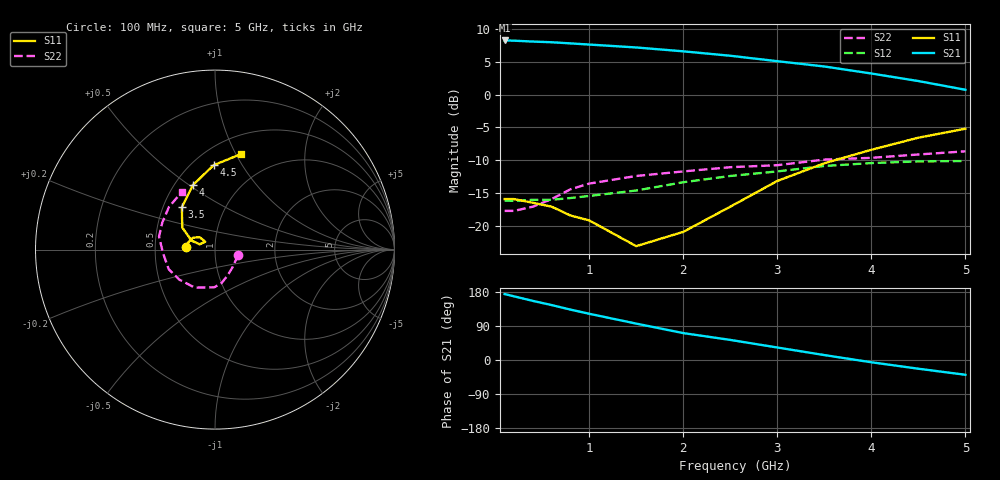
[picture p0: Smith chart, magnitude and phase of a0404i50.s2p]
!  MSA-0404 S AND NOISE PARAMETERS
!  Id=50mA  LAST UPDATED 07-22-92
# ghz s ma r 50
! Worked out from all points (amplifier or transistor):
!   14 points, 100 MHz to 5 GHz, reference 50 ohm
!   highest |S21| = 8.3 dB at 100 MHz (marker M1)
!   |S21| within 3 dB of that: start of sweep to 2.903 GHz
!   unconditionally stable (mu >= 1): start of sweep to end of sweep
!   at 400 MHz: K = 1.38, MAG = 8.4 dB, |S12| = -16.0 dB
!   at 2 GHz: K = 1.22, MAG = 7.1 dB, |S12| = -13.4 dB
!   at 5 GHz: K = 1.10, MAG = 3.5 dB, |S12| = -10.1 dB
!   lowest NFmin = 6.70 dB at 100 MHz
!   S11 on the Smith chart (normalised r, x): 100 MHz: 0.72, +0.02; 3.5 GHz: 0.62, +0.32; 4 GHz: 0.61, +0.52; 4.5 GHz: 0.63, +0.76; 5 GHz: 0.69, +1.04
0.1  0.16 175.0  2.59 174.0  0.156 0.0  0.13 -13.0
0.2  0.16 170.0  2.58 168.0  0.155 2.0  0.13 -25.0
0.4  0.15 161.0  2.54 156.0  0.158 4.0  0.14 -47.0
0.6  0.14 152.0  2.51 145.0  0.158 6.0  0.16 -64.0
0.8  0.12 145.0  2.46 133.0  0.163 8.0  0.19 -79.0
1  0.11 141.0  2.41 122.0  0.169 9.0  0.21 -91.0
1.5  0.07 141.0  2.29 96.0  0.186 13.0  0.24 -118.0
2  0.09 161.0  2.14 71.0  0.215 12.0  0.26 -140.0
2.5  0.14 159.0  1.98 53.0  0.24 13.0  0.28 -157.0
3  0.22 146.0  1.8 33.0  0.26 7.0  0.29 -176.0
3.5  0.3 128.0  1.64 13.0  0.286 0.0  0.32 167.0
4  0.38 109.0  1.45 -6.0  0.301 -7.0  0.33 153.0
4.5  0.47 91.0  1.27 -23.0  0.31 -15.0  0.35 137.0
5  0.55 75.0  1.09 -39.0  0.312 -24.0  0.37 120.0
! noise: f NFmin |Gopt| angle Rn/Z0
0.1  6.7  0.11  -178  0.68
0.5  6.7  0.12  -167  0.68
1  6.9  0.14  -153  0.69
2  7.6  0.2  -125  0.77
